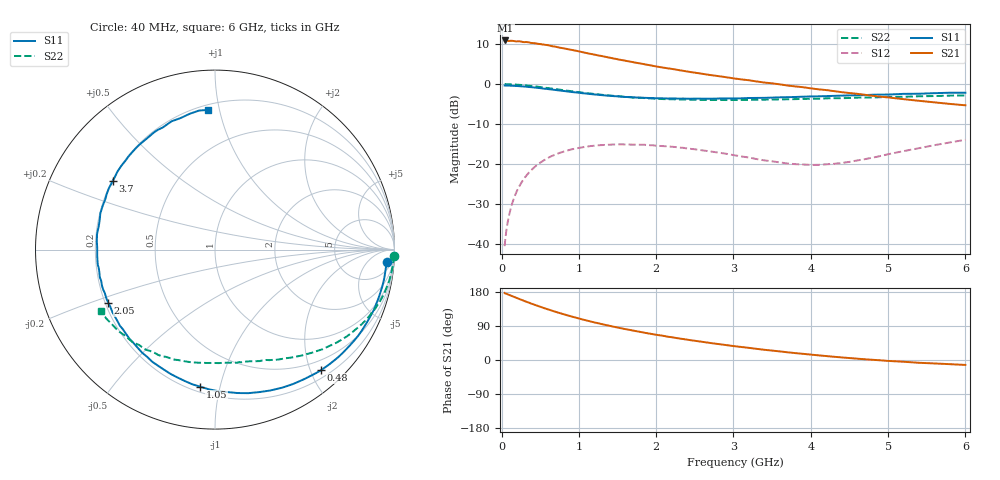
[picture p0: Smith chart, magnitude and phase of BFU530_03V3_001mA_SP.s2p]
! Filename:  P:\Prog\Test\Noise\ATS_data\Testdata_Net\03 Spar\BFU530_APG2013_40_A05_03p3V_001mA_SP_CM01_D.s2p
! Date/Time: Fri 26/Apr/2013 13:03:05
! BFU530_APG2013_40_A05_03p3V_1to25mA_SP_CM01_Bias1_R.s2p
! MDIF S-parameter v. bias file
! BFU530_APG2013_40_A05_03p3V_1to25mA_SP_CM01
! Date/time Wed Apr 24 18:17:07 2013
! bias mode 1
! bias variable = I_out
! VAR bias_var= 1
! VAR V_out= 3.3000
! VAR I_out= 0.9950
! VAR V_in= 0.7830
! VAR I_in= 0.0107
! Device data file deembeded for feedlines and parallel
! Original file: \03 Spar\BFU530_APG2013_40_A05_03p3V_001mA_SP_CM01_R.s2p
! Feed-files: PR047V01_250413_Feed1.s2p, PR047V01_250413_Feed2.s2p
! Parallel-file: PR047V01_250413_Par.s2p
# MHz S MA R 50
!  Freq-MHz  S11-mag  S11-arg  S21-mag  S21-arg  S12-mag  S12-arg  S22-mag  S22-arg
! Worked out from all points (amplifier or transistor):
!   98 points, 40 MHz to 6 GHz, reference 50 ohm
!   highest |S21| = 10.9 dB at 50 MHz (marker M1)
!   |S21| within 3 dB of that: start of sweep to 1.066 GHz
!   unconditionally stable (mu >= 1): 3.272 GHz to 5.104 GHz
!   at 300 MHz: K = 0.09, MSG = 16.9 dB, |S12| = -23.4 dB
!   at 1.6 GHz: K = 0.41, MSG = 10.5 dB, |S12| = -15.1 dB
!   at 6 GHz: K = 0.83, MSG = 4.3 dB, |S12| = -13.9 dB
!   S11 on the Smith chart (normalised r, x): 40 MHz: 12, -21; 480 MHz: 0.32, -2.18; 1.05 GHz: 0.23, -0.87; 2.05 GHz: 0.21, -0.23; 3.7 GHz: 0.20, +0.29; 6 GHz: 0.23, +0.93
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40  0.9596 -4.2  3.495 177.0  0.009472 87.0  0.9972 -2.0
50  0.9582 -5.2  3.503 175.3  0.01183 86.5  0.9989 -2.6
100  0.956 -10.3  3.45 171.7  0.02357 83.1  0.9937 -5.6
120  0.9544 -12.6  3.478 170.0  0.02821 81.8  0.9919 -6.8
200  0.9467 -20.7  3.406 163.4  0.04639 76.2  0.9819 -11.4
240  0.9395 -25.0  3.415 160.1  0.05509 73.5  0.9765 -13.6
340  0.9226 -35.0  3.327 152.3  0.07562 67.1  0.9556 -19.0
480  0.895 -48.6  3.169 142.0  0.1012 58.6  0.9229 -25.9
600  0.8663 -59.8  3.059 133.7  0.1194 51.9  0.8911 -31.4
700  0.8431 -68.7  2.926 127.1  0.1321 46.6  0.8649 -35.5
900  0.7972 -84.9  2.679 115.1  0.1527 37.5  0.8168 -42.8
1050  0.7682 -96.2  2.5 106.8  0.1626 31.3  0.7803 -47.9
1250  0.7352 -109.8  2.277 97.0  0.1721 24.2  0.745 -53.5
1500  0.7032 -125.3  2.041 85.7  0.1766 16.3  0.7058 -60.2
1750  0.6786 -139.1  1.839 75.8  0.1755 9.8  0.6753 -66.1
2050  0.6644 -153.5  1.628 65.1  0.1688 3.5  0.6515 -72.7
2500  0.6586 -172.6  1.389 50.8  0.1534 -3.3  0.6361 -82.1
3100  0.6638 165.2  1.145 34.4  0.125 -5.4  0.6335 -94.2
3700  0.686 146.1  0.9585 20.3  0.1019 3.2  0.6459 -106.4
4100  0.7032 135.2  0.8595 12.3  0.09813 15.2  0.6568 -114.5
5200  0.7547 108.7  0.648 -4.6  0.1456 37.1  0.6937 -136.3
6000  0.7796 92.8  0.5431 -13.0  0.2016 35.8  0.7221 -151.7
